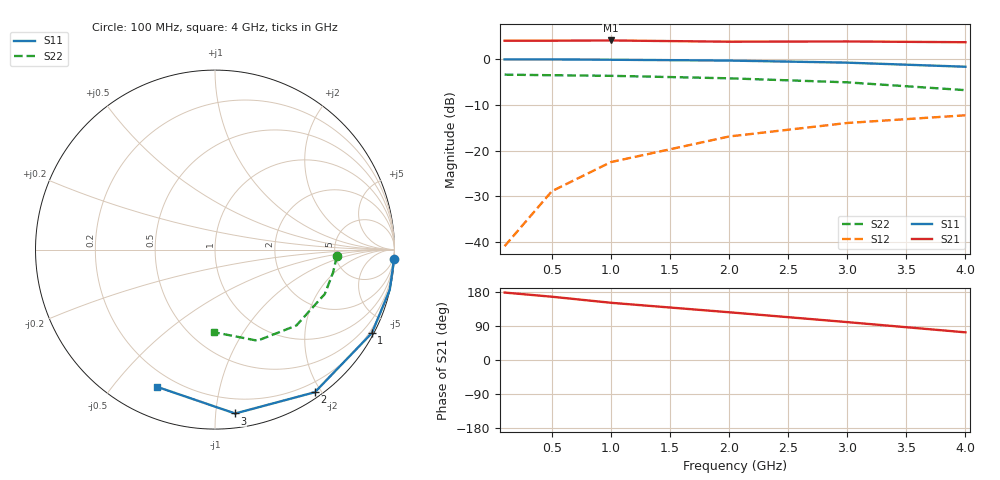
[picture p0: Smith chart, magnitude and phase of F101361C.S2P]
!ATF-10136
!S-PARAMETERS at Vds=1V  Id=2mA.  LAST UPDATED 06-29-94
# ghz s ma r 50
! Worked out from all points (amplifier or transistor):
!   6 points, 100 MHz to 4 GHz, reference 50 ohm
!   highest |S21| = 4.1 dB at 1 GHz (marker M1)
!   |S21| within 3 dB of that: start of sweep to end of sweep
!   unconditionally stable (mu >= 1): nowhere
!   at 500 MHz: K = 0.05, MSG = 16.5 dB, |S12| = -28.9 dB
!   at 2 GHz: K = 0.17, MSG = 10.4 dB, |S12| = -16.9 dB
!   at 4 GHz: K = 0.43, MSG = 8.0 dB, |S12| = -12.3 dB
!   lowest NFmin = 0.40 dB at 500 MHz
!   S11 on the Smith chart (normalised r, x): 100 MHz: 1, -38; 1 GHz: 0.09, -4.01; 2 GHz: 0.07, -1.92; 3 GHz: 0.09, -1.13; 4 GHz: 0.13, -0.65
0.1  0.999 -3.0  1.6 178.0  0.009 76.0  0.68 -3.0
0.5  0.999 -13.0  1.6 167.0  0.036 78.0  0.67 -11.0
1  0.99 -28.0  1.61 151.0  0.075 69.0  0.66 -22.0
2  0.97 -55.0  1.56 126.0  0.143 48.0  0.62 -43.0
3  0.92 -83.0  1.57 100.0  0.201 27.0  0.56 -65.0
4  0.83 -113.0  1.54 73.0  0.244 6.0  0.46 -91.0
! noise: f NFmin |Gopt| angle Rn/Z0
0.5  0.4  0.93  12  0.85
1  0.4  0.85  24  0.7
2  0.4  0.7  47  0.46
4  0.5  0.39  126  0.36
